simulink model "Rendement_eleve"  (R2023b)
settings: Solver=VariableStepAuto  StartTime=0.0  StopTime=10.0  RelTol=1e-3
model workspace (MAT data in the model file):
  rendement = 0.6
libraries: fl_lib x22, nesl_utility x7, ee_lib x2

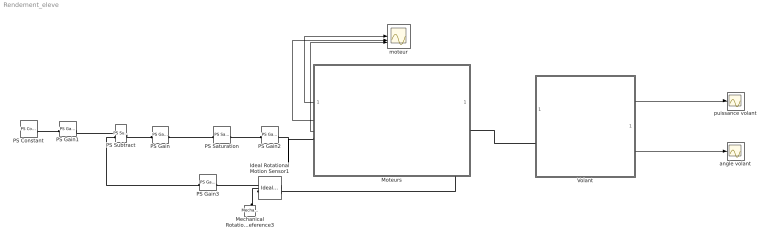
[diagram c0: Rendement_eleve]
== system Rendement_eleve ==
  Ideal Rotational Motion Sensor1 : fl_lib/Mechanical/Mechanical Sensors/Ideal Rotational Motion Sensor  reference=foundation.enum.MeasurementReference.difference  acceleration_port=false  velocity_port=false  position_port=true  wrap_angle=false  offset=0 rad
  Mechanical Rotational Reference3 : fl_lib/Mechanical/Rotational Elements/Mechanical Rotational Reference
  Moteurs : Subsystem  mask{Kc=0}
  PS Constant : fl_lib/Physical Signals/Sources/PS Constant  constant=0
  PS Gain : fl_lib/Physical Signals/Functions/PS Gain  gain=7
  PS Gain1 : fl_lib/Physical Signals/Functions/PS Gain  gain=120*11/(2*pi*180)
  PS Gain2 : fl_lib/Physical Signals/Functions/PS Gain  gain=24/1204
  PS Gain3 : fl_lib/Physical Signals/Functions/PS Gain  gain=120/(2*pi)
  PS Saturation : fl_lib/Physical Signals/Nonlinear Operators/PS Saturation  upper_limit=1024  lower_limit=-1024
  PS Subtract : fl_lib/Physical Signals/Functions/PS Subtract
  Volant : Subsystem  mask{rendement=0}
  angle volant : Scope
  moteur : Scope  NumInputPorts=3
  puissance volant : Scope
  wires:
  Moteurs/1(Out1) -> moteur/1
  Moteurs/2(Out2) -> moteur/2
  Moteurs/3(Out3) -> moteur/3
  Volant/1(Out1) -> puissance volant/1
  Volant/2(Out2) -> angle volant/1
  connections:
  Mechanical Rotational Reference3/LConn1 -- Ideal Rotational Motion Sensor1/RConn1
  Ideal Rotational Motion Sensor1/RConn2 -- PS Gain3/LConn1
  PS Gain/RConn1 -- PS Saturation/LConn1
  PS Saturation/RConn1 -- PS Gain2/LConn1
  PS Constant/RConn1 -- PS Gain1/LConn1
  PS Gain1/RConn1 -- PS Subtract/LConn1
  PS Subtract/RConn1 -- PS Gain/LConn1
  PS Subtract/LConn2 -- PS Gain3/RConn1
  PS Gain2/RConn1 -- Moteurs/RConn1
  Ideal Rotational Motion Sensor1/LConn1 -- Moteurs/LConn1 -- Volant/LConn1

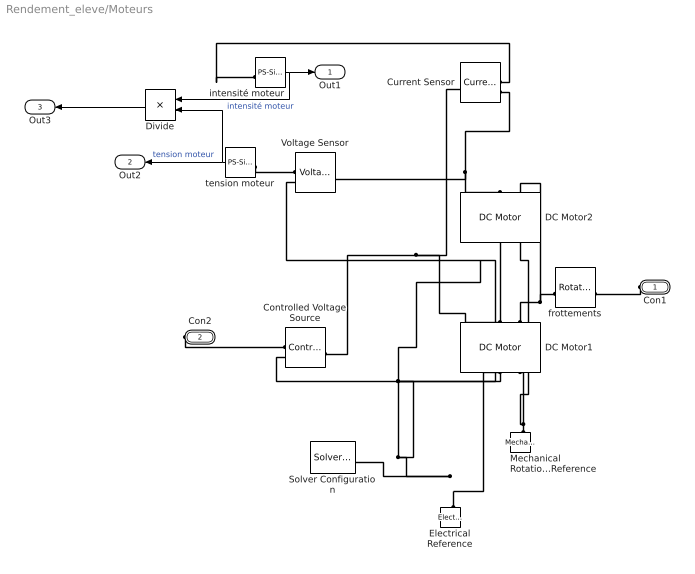
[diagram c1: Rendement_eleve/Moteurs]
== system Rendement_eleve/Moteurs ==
  Controlled Voltage Source : fl_lib/Electrical/Electrical Sources/Controlled Voltage Source
  Current Sensor : fl_lib/Electrical/Electrical Sensors/Current Sensor
  DC Motor1 : ee_lib/Electromechanical/Brushed Motors/DC Motor  field_option=ee.enum.field_option.pm  Rf=100 Ohm  Lf=1 H  Laf=0.15 H  If0=0 A  parameterization=ee.enum.dcparam_option.circuit_param  Ra=26 Ohm  La=0.001 H  emf_or_torque=ee.enum.emf_or_torque.ki  Kv=0.072e-3 V*s/rad  Ki=Kc N*m/A  T_stall=0.24e-3 N*m  w_max=19100 rpm  w_rated=15000 rpm  P_rated=0.08 W  V_rated=1.5 V  lam_param=ee.enum.lam_param.damping  i_noload=0 A  V_i_noload=1.5 V  J=2.5e-5 kg*m^2  lam=0 N*m*s/rad  speed0=0 rpm  enable_fault_armature=simscape.enum.onoff.off  rev_faulted=1 / 3  G_faulted_armature=1e-5 S  fault_trigger_armature=ee.enum.faults.faultTrigger.temporal  t_fault_armature=1 s  max_permissible_current_armature=inf A  t_fail_on_current_armature=1 s  enable_fault_field=simscape.enum.onoff.off  G_faulted_field=1e-5 S  fault_trigger_field=ee.enum.faults.faultTrigger.temporal  t_fault_field=1 s  max_permissible_current_field=inf A  t_fail_on_current_field=1 s  fault_action=simscape.enum.assert.action.none  alpha=3.93e-3 1/K  Tmeas=25 degC  thermal_mass=100 J/K  initial_temperature=25 degC
  DC Motor2 : ee_lib/Electromechanical/Brushed Motors/DC Motor  field_option=ee.enum.field_option.pm  Rf=100 Ohm  Lf=1 H  Laf=0.15 H  If0=0 A  parameterization=ee.enum.dcparam_option.circuit_param  Ra=26 Ohm  La=0.001 H  emf_or_torque=ee.enum.emf_or_torque.ki  Kv=0.072e-3 V*s/rad  Ki=Kc N*m/A  T_stall=0.24e-3 N*m  w_max=19100 rpm  w_rated=15000 rpm  P_rated=0.08 W  V_rated=1.5 V  lam_param=ee.enum.lam_param.damping  i_noload=0 A  V_i_noload=1.5 V  J=2.5e-5 kg*m^2  lam=0 N*m*s/rad  speed0=0 rpm  enable_fault_armature=simscape.enum.onoff.off  rev_faulted=1 / 3  G_faulted_armature=1e-5 S  fault_trigger_armature=ee.enum.faults.faultTrigger.temporal  t_fault_armature=1 s  max_permissible_current_armature=inf A  t_fail_on_current_armature=1 s  enable_fault_field=simscape.enum.onoff.off  G_faulted_field=1e-5 S  fault_trigger_field=ee.enum.faults.faultTrigger.temporal  t_fault_field=1 s  max_permissible_current_field=inf A  t_fail_on_current_field=1 s  fault_action=simscape.enum.assert.action.none  alpha=3.93e-3 1/K  Tmeas=25 degC  thermal_mass=100 J/K  initial_temperature=25 degC
  Divide : Product  Inputs=**
  Electrical Reference : fl_lib/Electrical/Electrical Elements/Electrical Reference
  Mechanical Rotational Reference : fl_lib/Mechanical/Rotational Elements/Mechanical Rotational Reference
  Solver Configuration : nesl_utility/Solver Configuration  PhysicalDomain=network_engine_domain  SubClassName=solver  LeftPortType=input  RightPortType=generic  Tones=[]  Harmonics=[]  SimulateNoise=off  Profile=off  UseLocalSampling=off  EnableSwitchedLinearOptims=on  FrequencyDomain=off  UseCCode=off  RelTol=0.001  AbsTol=0.001  MinStep=1e-09  ToWorkspace=off  RevertToSquareIcSolve=off  NumHomotopyIterations=100  PhasorMode=off  PhasorModeNumHarmonics=1  ConsistencySolver=NEWTON_XTOL_AFTER_FTOL  IndexReductionMethod=DerivativeReplacement  DoDC=off  ResidualTolerance=1e-09  ConsistencyTolSource=GLOBAL  ConsistencyAbsTol=0.001  ConsistencyRelTol=0.001  ConsistencyTolFactor=0.001  UseLocalSolver=on  LocalSolverChoice=NE_BACKWARD_EULER_ADVANCER  ResolveIndetEquations=on  FunctionEvalNumThread=1  LocalSolverSampleTime=0.001  DoFixedCost=on  MaxNonlinIter=3  MaxModeIter=2  ComputeImpulses=off  ImpulseIterations=2  LinearAlgebra=auto  LinearAlgebraNumThread=0  EquationFormulation=NE_TIME_EF  DelaysMemoryBudget=1024  AutomaticFiltering=on  FilteringTimeConstant=0.001  PartitionStorageMethod=AS_NEEDED  PartitionMemoryBudget=1024  PartitionMethod=ROBUST  MultibodyUseLocalSolver=on  MultibodyLocalSolverChoice=ODE1  MultibodyLocalSolverSampleTime=0.001
  Voltage Sensor : fl_lib/Electrical/Electrical Sensors/Voltage Sensor
  frottements : fl_lib/Mechanical/Rotational Elements/Rotational Friction  brkwy_trq=1 N*m  brkwy_vel=0.1 rad/s  Col_trq=16e-3 N*m  visc_coef=0.001 N*m*s/rad  w_specify=off  w_priority=None  w=0 rad/s  w_nominal_specify=off  w_nominal_unit=rad/s  w_nominal_value=1  t_specify=off  t_priority=None  t=0 N*m  t_nominal_specify=off  t_nominal_unit=N*m  t_nominal_value=1
  intensité moteur : nesl_utility/PS-Simulink Converter  PhysicalDomain=network_engine_domain  SubClassName=ps_output  LeftPortType=input  RightPortType=output  PseudoPeriodic=off  Frequencies=[]  VectorFormat=1-D array  Unit=1  AffineConversion=off
  tension moteur : nesl_utility/PS-Simulink Converter  PhysicalDomain=network_engine_domain  SubClassName=ps_output  LeftPortType=input  RightPortType=output  PseudoPeriodic=off  Frequencies=[]  VectorFormat=inherit  Unit=1  AffineConversion=off
  Con1 : PMIOPort  Side=Left
  Con2 : PMIOPort  Port=2  Side=Right
  Out1 : Outport
  Out2 : Outport  Port=2
  Out3 : Outport  Port=3
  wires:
  intensité moteur/1 -> Divide/1, Out1/1  "intensité moteur"
  tension moteur/1 -> Out2/1, Divide/2  "tension moteur"
  Divide/1 -> Out3/1
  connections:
  Con1/RConn1 -- frottements/RConn1
  Electrical Reference/LConn1 -- Voltage Sensor/RConn2 -- DC Motor2/RConn1 -- Controlled Voltage Source/RConn2 -- Solver Configuration/RConn1 -- DC Motor1/RConn1
  Mechanical Rotational Reference/LConn1 -- DC Motor2/RConn2 -- DC Motor1/RConn2
  Controlled Voltage Source/LConn1 -- Current Sensor/LConn1 -- DC Motor1/LConn1
  Con2/RConn1 -- Controlled Voltage Source/RConn1
  DC Motor1/LConn2 -- DC Motor2/LConn2 -- frottements/LConn1
  Current Sensor/RConn2 -- Voltage Sensor/LConn1 -- DC Motor2/LConn1
  Current Sensor/RConn1 -- intensité moteur/LConn1
  tension moteur/LConn1 -- Voltage Sensor/RConn1

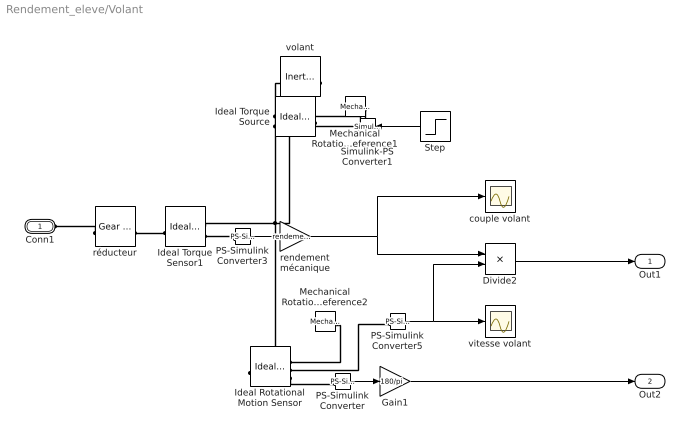
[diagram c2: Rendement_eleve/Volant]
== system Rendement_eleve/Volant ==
  Divide2 : Product  Inputs=**
  Gain1 : Gain  Gain=180/pi
  Ideal Rotational Motion Sensor : fl_lib/Mechanical/Mechanical Sensors/Ideal Rotational Motion Sensor  reference=foundation.enum.MeasurementReference.difference  acceleration_port=false  velocity_port=true  position_port=true  wrap_angle=false  offset=0 rad
  Ideal Torque Sensor1 : fl_lib/Mechanical/Mechanical Sensors/Ideal Torque Sensor
  Ideal Torque Source : fl_lib/Mechanical/Mechanical Sources/Ideal Torque Source
  Mechanical Rotational Reference1 : fl_lib/Mechanical/Rotational Elements/Mechanical Rotational Reference
  Mechanical Rotational Reference2 : fl_lib/Mechanical/Rotational Elements/Mechanical Rotational Reference
  PS-Simulink Converter : nesl_utility/PS-Simulink Converter  PhysicalDomain=network_engine_domain  SubClassName=ps_output  LeftPortType=input  RightPortType=output  PseudoPeriodic=off  Frequencies=[]  VectorFormat=inherit  Unit=inherit  AffineConversion=off
  PS-Simulink Converter3 : nesl_utility/PS-Simulink Converter  PhysicalDomain=network_engine_domain  SubClassName=ps_output  LeftPortType=input  RightPortType=output  PseudoPeriodic=off  Frequencies=[]  VectorFormat=inherit  Unit=inherit  AffineConversion=off
  PS-Simulink Converter5 : nesl_utility/PS-Simulink Converter  PhysicalDomain=network_engine_domain  SubClassName=ps_output  LeftPortType=input  RightPortType=output  PseudoPeriodic=off  Frequencies=[]  VectorFormat=inherit  Unit=inherit  AffineConversion=off
  Simulink-PS Converter1 : nesl_utility/Simulink-PS Converter  PhysicalDomain=network_engine_domain  SubClassName=ps_input  LeftPortType=input  RightPortType=output  PseudoPeriodic=off  Frequencies=[]  NoiseDistribution=none  NoiseParameters=[]  Unit=1  AffineConversion=off  FilteringAndDerivatives=provide  SimscapeFilterOrder=1  InputFilterTimeConstant=0.001  UdotUserProvided=0
  Step : Step  Time=0.3  Before=7  After=0  SampleTime=0
  couple volant : Scope
  rendement mécanique : Gain  Gain=rendement
  réducteur : fl_lib/Mechanical/Mechanisms/Gear Box  ratio=180/11  t_in_specify=off  t_in_priority=None  t_in=0 N*m  t_in_nominal_specify=off  t_in_nominal_unit=N*m  t_in_nominal_value=1  t_out_specify=off  t_out_priority=None  t_out=0 N*m  t_out_nominal_specify=off  t_out_nominal_unit=N*m  t_out_nominal_value=1
  vitesse volant : Scope
  volant : fl_lib/Mechanical/Rotational Elements/Inertia  inertia=0.011 kg*m^2  num_ports=foundation.enum.numPorts2.one  w_specify=off  w_priority=High  w=0 rad/s  w_nominal_specify=off  w_nominal_unit=rad/s  w_nominal_value=1  t_specify=off  t_priority=None  t=0 N*m  t_nominal_specify=off  t_nominal_unit=N*m  t_nominal_value=1
  Conn1 : PMIOPort  Side=Left
  Out1 : Outport
  Out2 : Outport  Port=2
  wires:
  Gain1/1 -> Out2/1
  Step/1 -> Simulink-PS Converter1/1
  PS-Simulink Converter5/1 -> Divide2/2, vitesse volant/1
  PS-Simulink Converter3/1 -> rendement mécanique/1
  PS-Simulink Converter/1 -> Gain1/1
  rendement mécanique/1 -> Divide2/1, couple volant/1
  Divide2/1 -> Out1/1
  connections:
  Ideal Torque Source/LConn1 -- Ideal Rotational Motion Sensor/LConn1 -- volant/LConn1 -- Ideal Torque Sensor1/RConn1
  Mechanical Rotational Reference2/LConn1 -- Ideal Rotational Motion Sensor/RConn1
  Mechanical Rotational Reference1/LConn1 -- Ideal Torque Source/RConn2
  Ideal Torque Sensor1/LConn1 -- réducteur/RConn1
  Simulink-PS Converter1/RConn1 -- Ideal Torque Source/RConn1
  PS-Simulink Converter5/LConn1 -- Ideal Rotational Motion Sensor/RConn2
  Ideal Rotational Motion Sensor/RConn3 -- PS-Simulink Converter/LConn1
  PS-Simulink Converter3/LConn1 -- Ideal Torque Sensor1/RConn2
  réducteur/LConn1 -- Conn1/RConn1
